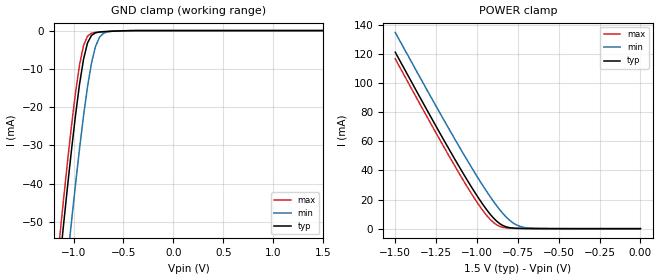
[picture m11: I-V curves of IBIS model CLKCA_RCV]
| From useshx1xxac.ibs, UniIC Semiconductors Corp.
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|   Model CLKCA_RCV
[Model]  CLKCA_RCV
Model_type   Input
Polarity   Non-Inverting
Vinl =   0.600000V
Vinh =   0.900000V
C_comp   0.9500pF   0.9400pF   0.9600pF
[Temperature Range]   25.0000   95.0000   0.0
[Voltage Range]   1.5000V   1.4000V   1.6000V
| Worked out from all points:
|   GND clamp passes 1 mA (typ) near -0.80 V on its own axis
|   POWER clamp passes 1 mA (typ) near -0.81 V on its own axis
[GND_clamp]
|Voltage   I(typ)   I(min)   I(max)
-1.5V     -160.2mA   -179.6mA   -153.6mA
-1.14V    -61.19mA   -80.68mA   -54.47mA
-1.1V     -50.85mA   -70.2mA    -44.19mA
-1.06V    -40.81mA   -59.91mA   -34.26mA
-1.02V    -31.17mA   -49.88mA   -24.86mA
-940mV    -14.08mA   -30.94mA   -9.019mA
-900mV    -7.546mA   -22.35mA   -3.942mA
-860mV    -3.248mA   -14.72mA   -1.471mA
-820mV    -1.257mA   -8.498mA   -679uA
-740mV    -379.1uA   -1.751mA   -362.1uA
-620mV    -174.8uA   -181.3uA   -197.1uA
1.5V      576.8pA    617.8pA    100.6pA
[POWER_clamp]
|Voltage   I(typ)   I(min)   I(max)
-1.5V     121.2mA    134.8mA    116.7mA
-1.18V    56.38mA    70.22mA    51.72mA
-1.08V    37.13mA    50.85mA    32.52mA
-1V       22.65mA    35.98mA    18.24mA
-940mV    12.9mA     25.44mA    8.994mA
-900mV    7.429mA    18.88mA    4.306mA
-860mV    3.386mA    12.92mA    1.531mA
-840mV    2.06mA     10.24mA    858.4uA
-800mV    675.4uA    5.743mA    318.3uA
-740mV    168.8uA    1.723mA    149uA
-660mV    60.96uA    258uA      88.02uA
0V        576.8pA    143pA      138.6pA
